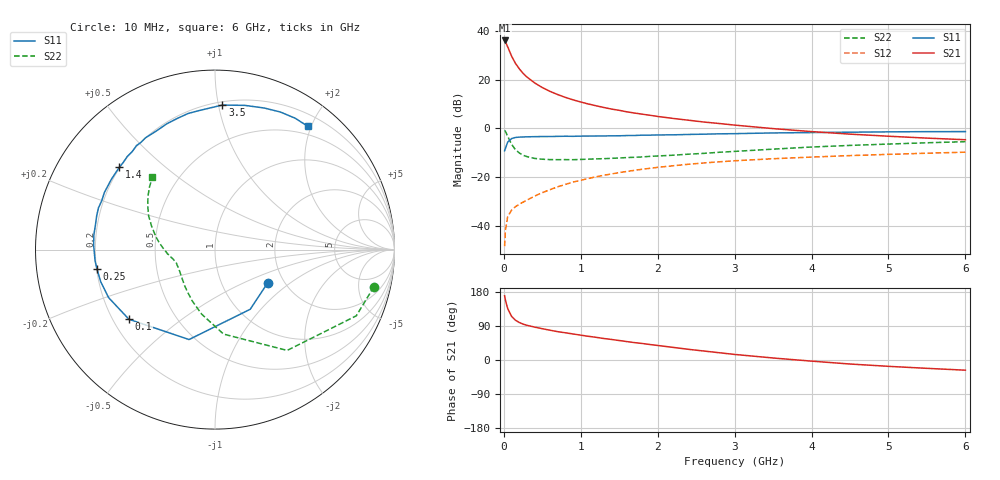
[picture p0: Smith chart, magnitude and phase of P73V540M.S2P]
! SIEMENS Small Signal Semiconductors
! BFP196
! Si NPN RF Bipolar Junction Transistor in SOT143
! VCE = 3.5 V  IC = 40 mA
! Common Emitter S-Parameters:  May  1996
# GHz  S  MA  R  50
!  f  S11  S21  S12  S22
! GHz  MAG  ANG  MAG  ANG  MAG  ANG  MAG  ANG
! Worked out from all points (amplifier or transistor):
!   36 points, 10 MHz to 6 GHz, reference 50 ohm
!   highest |S21| = 36.1 dB at 10 MHz (marker M1)
!   |S21| within 3 dB of that: start of sweep to 55.2 MHz
!   unconditionally stable (mu >= 1): 492.5 MHz to 4.222 GHz
!   at 250 MHz: K = 0.79, MSG = 26.5 dB, |S12| = -30.3 dB
!   at 1.4 GHz: K = 1.10, MAG = 11.4 dB, |S12| = -18.7 dB
!   at 6 GHz: K = 0.97, MSG = 2.6 dB, |S12| = -9.8 dB
!   S11 on the Smith chart (normalised r, x): 10 MHz: 1.65, -0.69; 100 MHz: 0.26, -0.33; 250 MHz: 0.20, -0.08; 1.4 GHz: 0.20, +0.36; 3.5 GHz: 0.22, +1.03; 6 GHz: 0.37, +1.95
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0.01  0.347 -32.2  64.08 169.4  0.0038 82.7  0.9096 -13.1
0.02  0.386 -59.4  60.42 158.5  0.0079 73.5  0.8694 -25.1
0.05  0.5216 -106.1  47.48 135.7  0.0153 54.7  0.6909 -54.4
0.1  0.6169 -141.0  30.68 115.4  0.0209 47.4  0.4732 -84.2
0.15  0.6504 -155.7  21.81 105.2  0.0245 47.0  0.3671 -101.7
0.2  0.6613 -164.2  16.82 99.0  0.0276 48.7  0.313 -113.9
0.25  0.6663 -170.5  13.51 94.7  0.0305 50.7  0.2803 -123.3
0.3  0.6711 -174.7  11.36 91.6  0.0335 54.1  0.2631 -129.9
0.4  0.6764 178.0  8.61 86.8  0.0407 56.6  0.2417 -140.0
0.5  0.6798 173.2  6.901 82.6  0.0477 58.6  0.2325 -146.9
0.6  0.6801 168.4  5.758 78.6  0.0551 59.9  0.2284 -151.6
0.7  0.6856 164.0  4.954 74.8  0.063 60.4  0.2275 -155.0
0.9  0.6872 156.7  3.861 68.7  0.0789 60.0  0.2274 -160.4
1.1  0.6943 149.4  3.168 62.5  0.0936 58.9  0.2332 -163.9
1.4  0.7033 139.2  2.493 54.2  0.1159 55.6  0.2421 -168.3
1.7  0.7146 130.2  2.065 45.8  0.1377 52.1  0.2547 -172.8
2.2  0.737 116.5  1.601 33.3  0.1706 45.0  0.2811 -179.5
2.8  0.773 101.2  1.26 19.2  0.2056 36.6  0.3229 170.7
3.5  0.8064 87.1  0.989 5.3  0.2379 26.9  0.3746 160.1
4.5  0.8352 70.8  0.762 -10.6  0.2759 15.1  0.4467 147.0
5.5  0.8576 58.6  0.631 -22.0  0.3089 4.3  0.5061 136.1
6  0.8597 53.1  0.585 -26.9  0.3243 -1.4  0.5332 130.8
